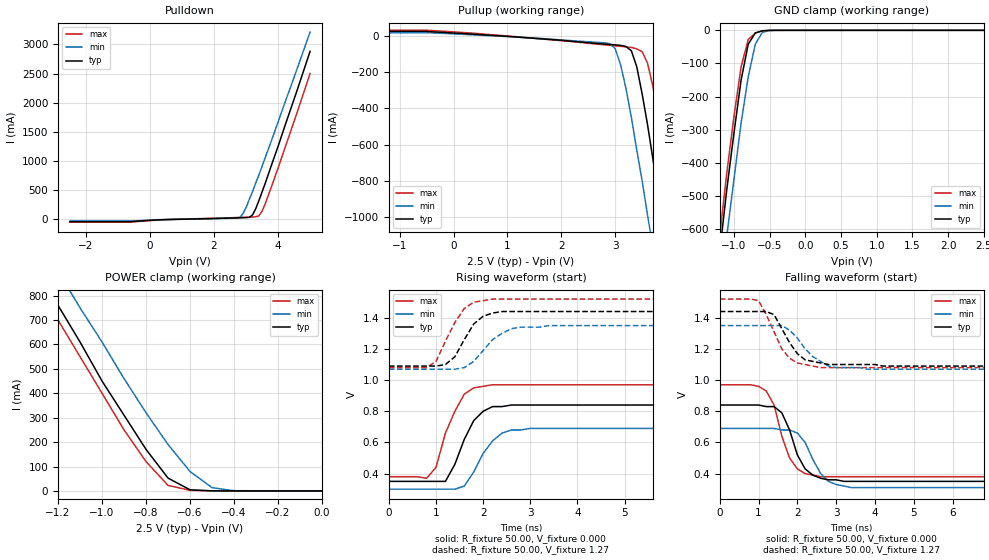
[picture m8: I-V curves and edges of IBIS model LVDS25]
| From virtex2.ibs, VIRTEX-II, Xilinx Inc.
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|   Model LVDS25
[Model]   LVDS25
Model_type   I/O
Polarity   Non-Inverting
Enable   Active-Low
Vinh = 1.4v
Vinl = 1.0v
Vmeas =   1.20V
Cref =  10.00pF
Rref =  50.00
Vref =   1.20V
C_comp   7.00pF   6.00pF   8.00pF
[Temperature Range]   25.00   100.00   0.000
[Voltage Range]   2.50V   2.30V   2.70V
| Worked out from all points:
|   slope of the pulldown table from 0 to 0.375 V, typ, clamps not added: 36.4 ohm
|   slope of the pullup table from 0 to 0.375 V, typ, clamps not added: 56.3 ohm
|   GND clamp passes 1 mA (typ) near -0.57 V on its own axis
|   POWER clamp passes 1 mA (typ) near -0.52 V on its own axis
|   rising waveform, R_fixture 50.00, V_fixture 0.000: 20-80 % time 428ps typ, 479ps min, 442ps max; typ from 0.35 V to 0.84 V
|   rising waveform, R_fixture 50.00, V_fixture 1.27: 20-80 % time 422ps typ, 553ps min, 464ps max; typ from 1.09 V to 1.44 V
|   falling waveform, R_fixture 50.00, V_fixture 0.000: 20-80 % time 473ps typ, 528ps min, 432ps max; typ from 0.84 V to 0.35 V
|   falling waveform, R_fixture 50.00, V_fixture 1.27: 20-80 % time 539ps typ, 656ps min, 533ps max; typ from 1.44 V to 1.09 V
[Pulldown]
| voltage   I(typ)   I(min)   I(max)
-2.5V     -40.4mA    -28.49mA   -48.63mA
-700mV    -40.4mA    -28.49mA   -48.63mA
2.8V      26.93mA    32.95mA    32.89mA
2.9V      28.43mA    94.12mA    34.57mA
3V        30.09mA    200mA      36.23mA
3.1V      34.6mA     340mA      37.89mA
3.2V      74.59mA    470mA      39.89mA
3.4V      320mA      760mA      60.32mA
3.5V      470mA      910mA      140mA
3.6V      620mA      1.06A      270mA
4V        1.25A      1.67A      880mA
5V        2.88A      3.21A      2.5A
[Pullup]
| voltage   I(typ)   I(min)   I(max)
-2.5V     24.97mA    16.95mA    32.29mA
-500mV    24.54mA    16.95mA    31.61mA
2.9V      -47mA      -42.9mA    -52.01mA
3V        -49.22mA   -69.62mA   -54.76mA
3.1V      -52.1mA    -160mA     -57.44mA
3.3V      -81.76mA   -450mA     -63.61mA
3.4V      -170mA     -630mA     -71.3mA
3.6V      -490mA     -990mA     -150mA
3.8V      -870mA     -1.36A     -450mA
4V        -1.27A     -1.74A     -830mA
4.2V      -1.68A     -2.13A     -1.22A
5V        -3.35A     -3.69A     -2.88A
[GND_clamp]
| voltage   I(typ)   I(min)   I(max)
-2.5V     -3.34A     -3.3A      -3.3A
-1.2V     -670mA     -800mA     -620mA
-1.1V     -480mA     -620mA     -430mA
-1V       -310mA     -450mA     -260mA
-900mV    -150mA     -280mA     -110mA
-800mV    -41.81mA   -140mA     -27.69mA
-700mV    -7.62mA    -40.98mA   -8.11mA
-600mV    -1.38mA    -5.69mA    -1.55mA
-500mV    -120uA     -670uA     -110uA
2.5V      540pA      2.11uA     480pA
[POWER_clamp]
| voltage   I(typ)   I(min)   I(max)
-2.5V     2.86A      2.89A      2.8A
-1.3V     920mA      1.05A      860mA
-1.2V     760mA      900mA      700mA
-1.1V     610mA      750mA      550mA
-1V       450mA      610mA      400mA
-900mV    310mA      460mA      250mA
-800mV    170mA      320mA      120mA
-700mV    52.5mA     190mA      22.73mA
-600mV    4.56mA     79.5mA     2.44mA
-500mV    270uA      13.41mA    250uA
-400mV    16.38uA    820uA      14.45uA
0V        540pA      2.08nA     580pA
[Ramp]
| variable   typ   min   max
dV/dt_r   0.29/0.41n   0.23/0.46n   0.35/0.35n
dV/dt_f   0.12/0.19n   90.00m/0.22n   0.17/0.18n
R_load = 50.00
[Rising Waveform]
R_fixture = 50.00
V_fixture = 0.000
| time   V(typ)   V(min)   V(max)
0s        350mV      300mV      380mV
800ps     350mV      300mV      370mV
1ns       350mV      300mV      440mV
1.2ns     350mV      300mV      660mV
1.4ns     460mV      300mV      800mV
1.6ns     620mV      320mV      910mV
1.8ns     740mV      410mV      950mV
2.2ns     830mV      610mV      970mV
2.6ns     840mV      680mV      970mV
10ns      840mV      690mV      970mV
[Rising Waveform]
R_fixture = 50.00
V_fixture = 1.27
V_fixture_min = 1.21
V_fixture_max = 1.30
| time   V(typ)   V(min)   V(max)
0s        1.09V      1.07V      1.08V
800ps     1.09V      1.07V      1.08V
1ns       1.09V      1.07V      1.12V
1.2ns     1.1V       1.07V      1.25V
1.6ns     1.26V      1.08V      1.46V
1.8ns     1.36V      1.12V      1.5V
2.2ns     1.43V      1.26V      1.52V
2.6ns     1.44V      1.33V      1.52V
3.4ns     1.44V      1.35V      1.52V
10ns      1.44V      1.35V      1.52V
[Falling Waveform]
R_fixture = 50.00
V_fixture = 0.000
| time   V(typ)   V(min)   V(max)
0s        840mV      690mV      970mV
1.2ns     830mV      690mV      930mV
1.4ns     830mV      690mV      840mV
1.6ns     790mV      680mV      640mV
1.8ns     680mV      680mV      500mV
2ns       520mV      660mV      430mV
2.2ns     430mV      600mV      400mV
2.8ns     360mV      350mV      380mV
3.4ns     350mV      310mV      380mV
10ns      350mV      300mV      380mV
[Falling Waveform]
R_fixture = 50.00
V_fixture = 1.27
V_fixture_min = 1.21
V_fixture_max = 1.30
| time   V(typ)   V(min)   V(max)
0s        1.44V      1.35V      1.52V
1ns       1.44V      1.35V      1.51V
1.4ns     1.42V      1.35V      1.31V
1.6ns     1.33V      1.35V      1.2V
1.8ns     1.24V      1.32V      1.14V
2.2ns     1.13V      1.2V       1.1V
2.6ns     1.11V      1.12V      1.08V
3ns       1.1V       1.08V      1.08V
3.8ns     1.1V       1.07V      1.08V
10ns      1.09V      1.07V      1.08V
